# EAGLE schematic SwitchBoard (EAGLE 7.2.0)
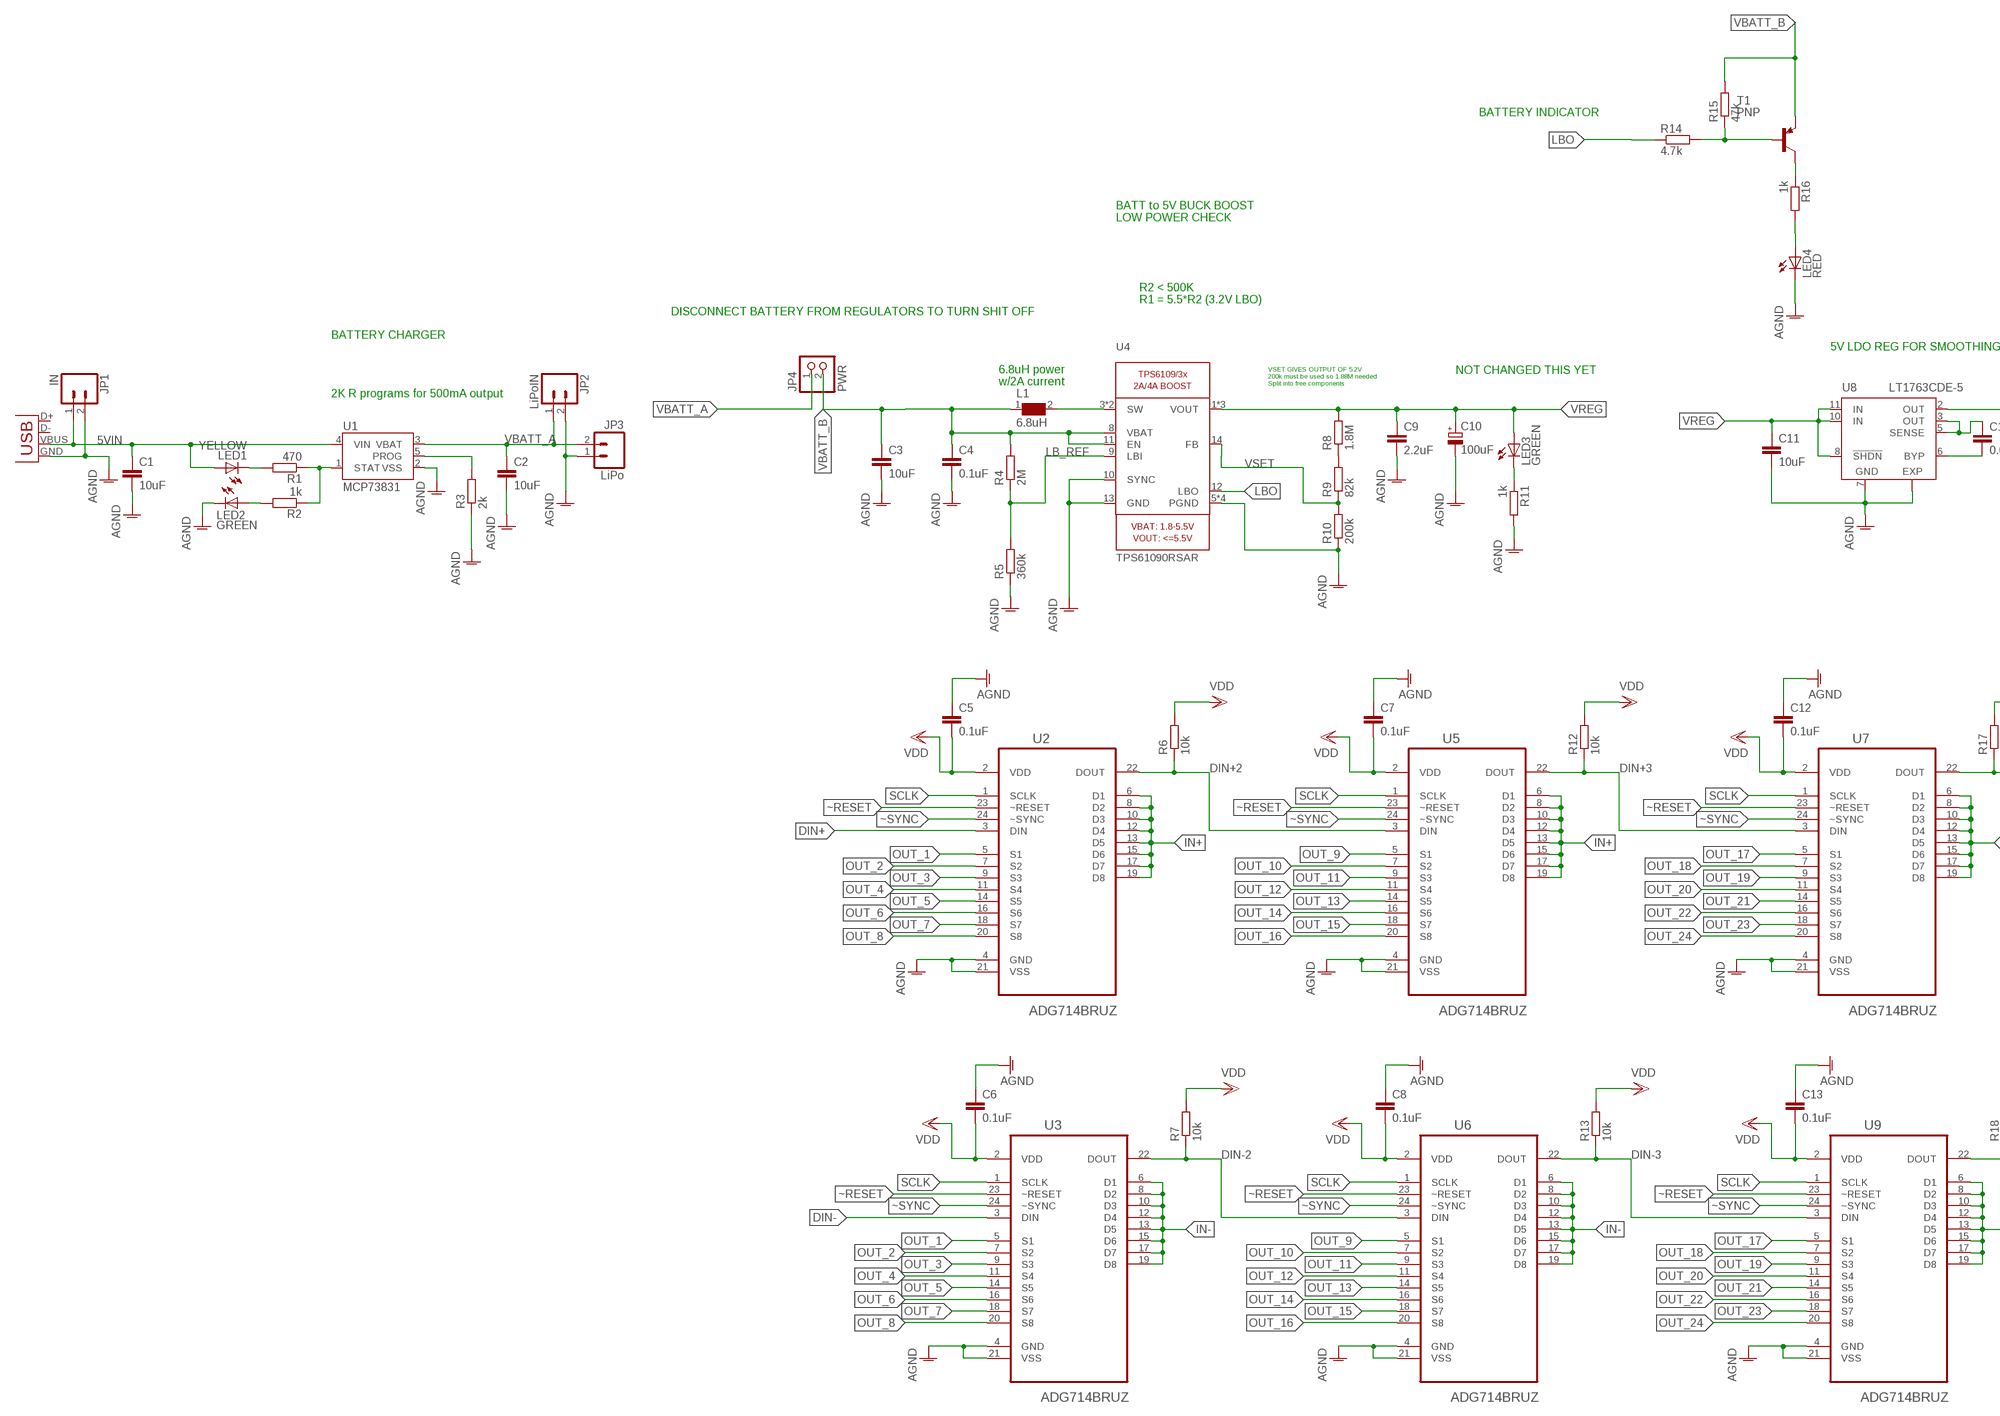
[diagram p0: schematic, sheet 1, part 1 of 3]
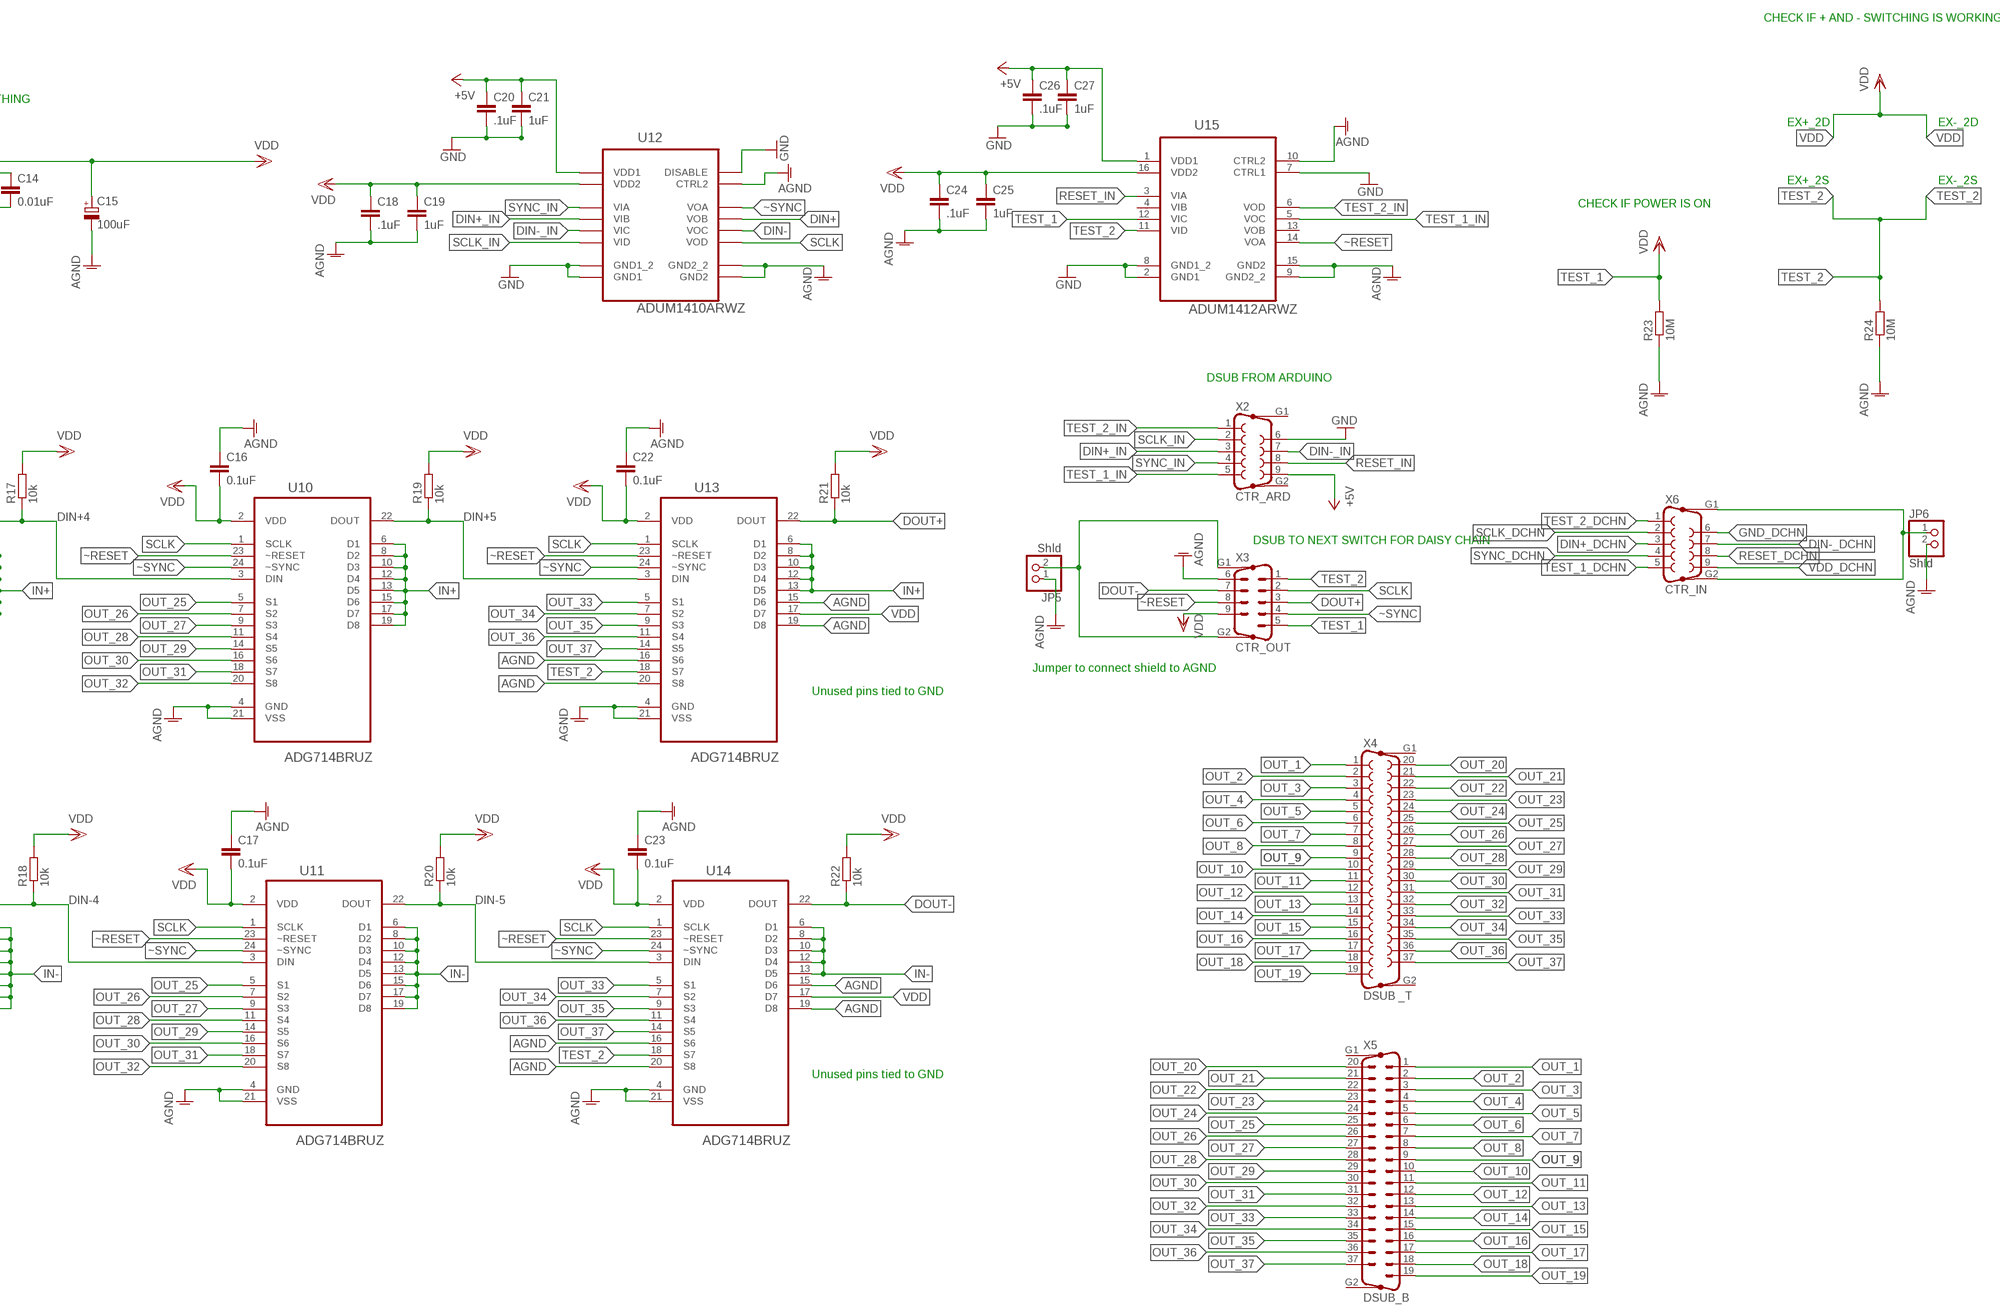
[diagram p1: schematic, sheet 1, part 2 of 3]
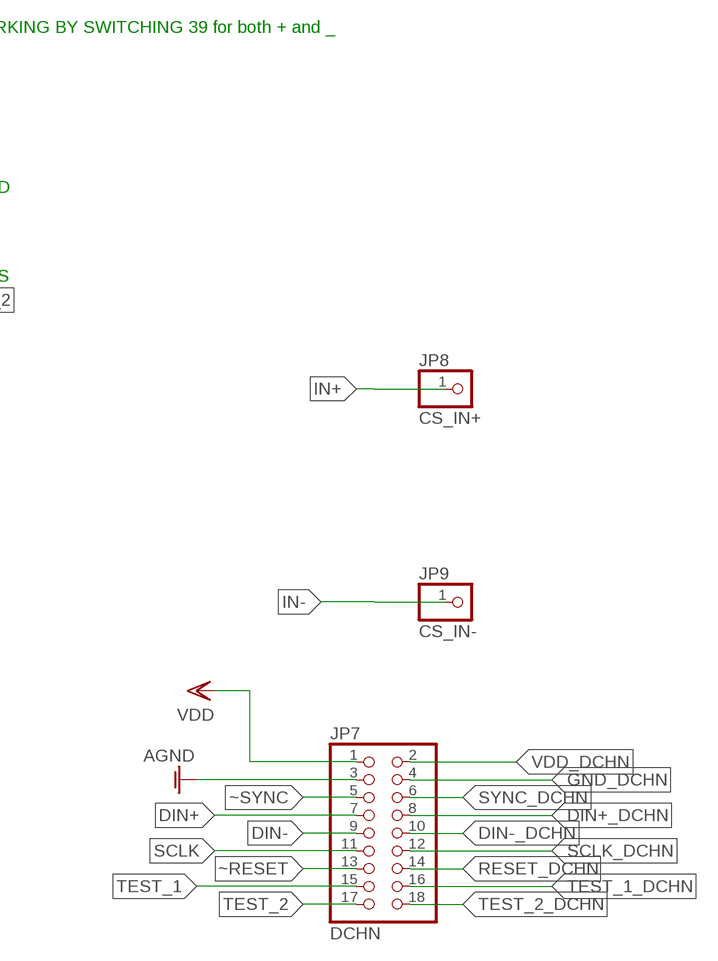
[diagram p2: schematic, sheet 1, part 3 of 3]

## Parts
C1  10uF  C-EUC0805  [C0805]
C2  10uF  C-EUC0805  [C0805]
C3  10uF  C-EUC0805  [C0805]
C4  0.1uF  C-EUC0805  [C0805]
C5  0.1uF  C-EUC0805  [C0805]
C6  0.1uF  C-EUC0805  [C0805]
C7  0.1uF  C-EUC0805  [C0805]
C8  0.1uF  C-EUC0805  [C0805]
C9  2.2uF  C-EUC0805  [C0805]
C10  100uF  CPOL-EUCT6032  [CT6032]
C11  10uF  C-EUC0805  [C0805]
C12  0.1uF  C-EUC0805  [C0805]
C13  0.1uF  C-EUC0805  [C0805]
C14  0.01uF  C-EUC0805  [C0805]
C15  100uF  CPOL-EUCT6032  [CT6032]
C16  0.1uF  C-EUC0805  [C0805]
C17  0.1uF  C-EUC0805  [C0805]
C18  .1uF  C-EUC0805  [C0805]
C19  1uF  C-EUC0805  [C0805]
C20  .1uF  C-EUC0805  [C0805]
C21  1uF  C-EUC0805  [C0805]
C22  0.1uF  C-EUC0805  [C0805]
C23  0.1uF  C-EUC0805  [C0805]
C24  .1uF  C-EUC0805  [C0805]
C25  1uF  C-EUC0805  [C0805]
C26  .1uF  C-EUC0805  [C0805]
C27  1uF  C-EUC0805  [C0805]
JP1  IN  M02PTH  [1X02]
JP2  LiPoIN  M02PTH  [1X02]
JP3  LiPo  M02-JST-2MM-SMT  [JST-2-SMD]
JP4  PWR  PINHD-1X2  [1X02]
JP5  Shld  PINHD-1X2  [1X02]
JP6  Shld  PINHD-1X2  [1X02]
JP7  DCHN  PINHD-2X9  [2X09]
JP8  CS_IN+  PINHD-1X1  [1X01]
JP9  CS_IN-  PINHD-1X1  [1X01]
L1  6.8uH  WE-PD-7447779006_7332/7345_PLASTIC_BASE  [WE-PD_7332/7345_PLASTIC_BASE]
LED1  YELLOW  LEDSML0805  [SML0805]
LED2  GREEN  LEDSML0805  [SML0805]
LED3  GREEN  LEDSML0805  [SML0805]
LED4  RED  LEDSML0805  [SML0805]
R1  470  R-EU_M0805  [M0805]
R2  1k  R-EU_M0805  [M0805]
R3  2k  R-EU_M0805  [M0805]
R4  2M  R-EU_M0805  [M0805]
R5  360k  R-EU_M0805  [M0805]
R6  10k  R-EU_M0805  [M0805]
R7  10k  R-EU_M0805  [M0805]
R8  1.8M  R-EU_M0805  [M0805]
R9  82k  R-EU_M0805  [M0805]
R10  200k  R-EU_M0805  [M0805]
R11  1k  R-EU_M0805  [M0805]
R12  10k  R-EU_M0805  [M0805]
R13  10k  R-EU_M0805  [M0805]
R14  4.7k  R-EU_M0805  [M0805]
R15  47k  R-EU_M0805  [M0805]
R16  1k  R-EU_M0805  [M0805]
R17  10k  R-EU_M0805  [M0805]
R18  10k  R-EU_M0805  [M0805]
R19  10k  R-EU_M0805  [M0805]
R20  10k  R-EU_M0805  [M0805]
R21  10k  R-EU_M0805  [M0805]
R22  10k  R-EU_M0805  [M0805]
R23  10M  R-EU_M0805  [M0805]
R24  10M  R-EU_M0805  [M0805]
T1  PNP  BC807-40-PNP-SOT23-BEC  [SOT23-BEC]
U1  MCP73831  [SOT23-5]
U2  ADG714BRUZ  [SOP65P640X120-24N]
U3  ADG714BRUZ  [SOP65P640X120-24N]
U4  TPS61090RSAR  VREG_TPS6103XSPARKFUNVERSION  [QFN16-4X4]
U5  ADG714BRUZ  [SOP65P640X120-24N]
U6  ADG714BRUZ  [SOP65P640X120-24N]
U7  ADG714BRUZ  [SOP65P640X120-24N]
U8  LT1763CDE-5  [DFN12]
U9  ADG714BRUZ  [SOP65P640X120-24N]
U10  ADG714BRUZ  [SOP65P640X120-24N]
U11  ADG714BRUZ  [SOP65P640X120-24N]
U12  ADUM1410ARWZ  [SOIC127P1032X265-16N]
U13  ADG714BRUZ  [SOP65P640X120-24N]
U14  ADG714BRUZ  [SOP65P640X120-24N]
U15  ADUM1412ARWZ  [SOIC127P1032X265-16N]
X1  USB-MICROB  [USB-MICROB]
X2  CTR_ARD  F09HP  [F09HP]
X3  CTR_OUT  M09HP  [M09HP]
X4  DSUB _T  F37HP  [F37HP]
X5  DSUB_B  M37HP  [M37HP]
X6  CTR_IN  F09HP  [F09HP]

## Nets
5VIN: C1.1 JP1.1 LED1.A U1.4(VIN) X1.VBUS
+5V: C20.1 C21.1 C26.1 C27.1 U12.1(VDD1) U15.1(VDD1) X2.9
AGND: C1.2 C2.2 C3.2 C4.2 C5.1 C6.1 C7.1 C8.1 C9.2 C10.- C11.2 C12.1 C13.1 C15.- C16.1 C17.1 C18.2 C19.2 C22.1 C23.1 C24.2 C25.2 JP1.2 JP2.2 JP3.1 JP5.1 JP6.2 JP7.3 LED2.C LED4.C R3.1 R5.1 R10.1 R11.2 R23.1 R24.1 U1.2(VSS) U2.4(GND) U2.21(VSS) U3.4(GND) U3.21(VSS) U4.5(PGND) U4.6(PGND) U4.7(PGND) U4.10(SYNC) U4.13(GND) U4.EXP(PGND) U5.4(GND) U5.21(VSS) U6.4(GND) U6.21(VSS) U7.4(GND) U7.21(VSS) U8.7(GND) U8.EXP U9.4(GND) U9.21(VSS) U10.4(GND) U10.21(VSS) U11.4(GND) U11.21(VSS) U12.9(GND2_2) U12.10(CTRL2) U12.15(GND2) U13.4(GND) U13.15(D6) U13.16(S6) U13.19(D8) U13.20(S8) U13.21(VSS) U14.4(GND) U14.15(D6) U14.16(S6) U14.19(D8) U14.20(S8) U14.21(VSS) U15.9(GND2_2) U15.10(CTRL2) U15.15(GND2) X1.GND X3.6
CHRG: LED1.C R1.2
DIN+: JP7.7 U2.3(DIN) U12.13(VOB)
DIN+2: R6.1 U2.22(DOUT) U5.3(DIN)
DIN+3: R12.1 U5.22(DOUT) U7.3(DIN)
DIN+4: R17.1 U7.22(DOUT) U10.3(DIN)
DIN+5: R19.1 U10.22(DOUT) U13.3(DIN)
DIN+_DCHN: JP7.8 X6.3
DIN+_IN: U12.4(VIB) X2.3
DIN-: JP7.9 U3.3(DIN) U12.12(VOC)
DIN-2: R7.1 U3.22(DOUT) U6.3(DIN)
DIN-3: R13.1 U6.22(DOUT) U9.3(DIN)
DIN-4: R18.1 U9.22(DOUT) U11.3(DIN)
DIN-5: R20.1 U11.22(DOUT) U14.3(DIN)
DIN-_DCHN: JP7.10 X6.7
DIN-_IN: U12.5(VIC) X2.7
DOUT+: R21.1 U13.22(DOUT) X3.3
DOUT-: R22.1 U14.22(DOUT) X3.7
GND: C20.2 C21.2 C26.2 C27.2 U12.2(GND1_2) U12.7(DISABLE) U12.8(GND1) U15.2(GND1) U15.7(CTRL1) U15.8(GND1_2) X2.6
GND_DCHN: JP7.4 X6.6
IN+: JP8.1 U2.6(D1) U2.8(D2) U2.10(D3) U2.12(D4) U2.13(D5) U2.15(D6) U2.17(D7) U2.19(D8) U5.6(D1) U5.8(D2) U5.10(D3) U5.12(D4) U5.13(D5) U5.15(D6) U5.17(D7) U5.19(D8) U7.6(D1) U7.8(D2) U7.10(D3) U7.12(D4) U7.13(D5) U7.15(D6) U7.17(D7) U7.19(D8) U10.6(D1) U10.8(D2) U10.10(D3) U10.12(D4) U10.13(D5) U10.15(D6) U10.17(D7) U10.19(D8) U13.6(D1) U13.8(D2) U13.10(D3) U13.12(D4) U13.13(D5)
IN-: JP9.1 U3.6(D1) U3.8(D2) U3.10(D3) U3.12(D4) U3.13(D5) U3.15(D6) U3.17(D7) U3.19(D8) U6.6(D1) U6.8(D2) U6.10(D3) U6.12(D4) U6.13(D5) U6.15(D6) U6.17(D7) U6.19(D8) U9.6(D1) U9.8(D2) U9.10(D3) U9.12(D4) U9.13(D5) U9.15(D6) U9.17(D7) U9.19(D8) U11.6(D1) U11.8(D2) U11.10(D3) U11.12(D4) U11.13(D5) U11.15(D6) U11.17(D7) U11.19(D8) U14.6(D1) U14.8(D2) U14.10(D3) U14.12(D4) U14.13(D5)
LB_REF: R4.1 R5.2 U4.9(LBI)
LBO: R14.1 U4.12(LBO)
N$3: C14.1 U8.3(OUT) U8.5(SENSE)
N$4: C14.2 U8.6(BYP)
N$5: LED2.A R2.2
N$6: R8.1 R9.2
N$7: LED3.C R11.1
N$8: R16.1 T1.C
N$9: LED4.A R16.2
N$10: JP5.2 X3.G1 X3.G2
N$11: R14.2 R15.1 T1.B
N$12: JP6.1 X6.G1 X6.G2
OUT_1: U2.5(S1) U3.5(S1) X4.1 X5.1
OUT_2: U2.7(S2) U3.7(S2) X4.2 X5.2
OUT_3: U2.9(S3) U3.9(S3) X4.3 X5.3
OUT_4: U2.11(S4) U3.11(S4) X4.4 X5.4
OUT_5: U2.14(S5) U3.14(S5) X4.5 X5.5
OUT_6: U2.16(S6) U3.16(S6) X4.6 X5.6
OUT_7: U2.18(S7) U3.18(S7) X4.7 X5.7
OUT_8: U2.20(S8) U3.20(S8) X4.8 X5.8
OUT_9: U5.5(S1) U6.5(S1) X4.9 X5.9
OUT_10: U5.7(S2) U6.7(S2) X4.10 X5.10
OUT_11: U5.9(S3) U6.9(S3) X4.11 X5.11
OUT_12: U5.11(S4) U6.11(S4) X4.12 X5.12
OUT_13: U5.14(S5) U6.14(S5) X4.13 X5.13
OUT_14: U5.16(S6) U6.16(S6) X4.14 X5.14
OUT_15: U5.18(S7) U6.18(S7) X4.15 X5.15
OUT_16: U5.20(S8) U6.20(S8) X4.16 X5.16
OUT_17: U7.5(S1) U9.5(S1) X4.17 X5.17
OUT_18: U7.7(S2) U9.7(S2) X4.18 X5.18
OUT_19: U7.9(S3) U9.9(S3) X4.19 X5.19
OUT_20: U7.11(S4) U9.11(S4) X4.20 X5.20
OUT_21: U7.14(S5) U9.14(S5) X4.21 X5.21
OUT_22: U7.16(S6) U9.16(S6) X4.22 X5.22
OUT_23: U7.18(S7) U9.18(S7) X4.23 X5.23
OUT_24: U7.20(S8) U9.20(S8) X4.24 X5.24
OUT_25: U10.5(S1) U11.5(S1) X4.25 X5.25
OUT_26: U10.7(S2) U11.7(S2) X4.26 X5.26
OUT_27: U10.9(S3) U11.9(S3) X4.27 X5.27
OUT_28: U10.11(S4) U11.11(S4) X4.28 X5.28
OUT_29: U10.14(S5) U11.14(S5) X4.29 X5.29
OUT_30: U10.16(S6) U11.16(S6) X4.30 X5.30
OUT_31: U10.18(S7) U11.18(S7) X4.31 X5.31
OUT_32: U10.20(S8) U11.20(S8) X4.32 X5.32
OUT_33: U13.5(S1) U14.5(S1) X4.33 X5.33
OUT_34: U13.7(S2) U14.7(S2) X4.34 X5.34
OUT_35: U13.9(S3) U14.9(S3) X4.35 X5.35
OUT_36: U13.11(S4) U14.11(S4) X4.36 X5.36
OUT_37: U13.14(S5) U14.14(S5) X4.37 X5.37
PROG: R3.2 U1.5(PROG)
RESET_DCHN: JP7.14 X6.8
RESET_IN: U15.3(VIA) X2.8
SCLK: JP7.11 U2.1(SCLK) U3.1(SCLK) U5.1(SCLK) U6.1(SCLK) U7.1(SCLK) U9.1(SCLK) U10.1(SCLK) U11.1(SCLK) U12.11(VOD) U13.1(SCLK) U14.1(SCLK) X3.2
SCLK_DCHN: JP7.12 X6.2
SCLK_IN: U12.6(VID) X2.2
STAT: R1.1 R2.1 U1.1(STAT)
SW: L1.2 U4.3(SW) U4.4(SW)
SYNC_DCHN: JP7.6 X6.4
SYNC_IN: U12.3(VIA) X2.4
TEST_1: JP7.15 R23.2 U15.12(VIC) X3.5 ; supply symbol labelled VDD
TEST_1_DCHN: JP7.16 X6.5
TEST_1_IN: U15.5(VOC) X2.5
TEST_2: JP7.17 R24.2 U13.18(S7) U14.18(S7) U15.11(VID) X3.1
TEST_2_DCHN: JP7.18 X6.1
TEST_2_IN: U15.6(VOD) X2.1
VBATT_A: C2.1 JP2.1 JP3.2 JP4.1 U1.3(VBAT)
VBATT_B: C3.1 C4.1 JP4.2 L1.1 R4.2 R15.2 T1.E U4.8(VBAT) U4.11(EN)
VDD: C5.2 C6.2 C7.2 C8.2 C12.2 C13.2 C15.+ C16.2 C17.2 C18.1 C19.1 C22.2 C23.2 C24.1 C25.1 JP7.1 R6.2 R7.2 R12.2 R13.2 R17.2 R18.2 R19.2 R20.2 R21.2 R22.2 U2.2(VDD) U3.2(VDD) U5.2(VDD) U6.2(VDD) U7.2(VDD) U8.2(OUT) U9.2(VDD) U10.2(VDD) U11.2(VDD) U12.16(VDD2) U13.2(VDD) U13.17(D7) U14.2(VDD) U14.17(D7) U15.16(VDD2) X3.9
VDD_DCHN: JP7.2 X6.9
VREG: C9.1 C10.+ C11.1 LED3.A R8.2 U4.1(VOUT) U4.15(VOUT) U4.16(VOUT) U8.8(!SHDN) U8.10(IN) U8.11(IN)
VSET: R9.1 R10.2 U4.14(FB)
~RESET: JP7.13 U2.23(~RESET) U3.23(~RESET) U5.23(~RESET) U6.23(~RESET) U7.23(~RESET) U9.23(~RESET) U10.23(~RESET) U11.23(~RESET) U13.23(~RESET) U14.23(~RESET) U15.14(VOA) X3.8
~SYNC: JP7.5 U2.24(~SYNC) U3.24(~SYNC) U5.24(~SYNC) U6.24(~SYNC) U7.24(~SYNC) U9.24(~SYNC) U10.24(~SYNC) U11.24(~SYNC) U12.14(VOA) U13.24(~SYNC) U14.24(~SYNC) X3.4
Unconnected: U15.4(VIB) U15.13(VOB) X1.D+ X1.D- X2.G1 X2.G2 X4.G1 X4.G2 X5.G1 X5.G2

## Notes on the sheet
- BATTERY INDICATOR
- BATT to 5V BUCK BOOST
  LOW POWER CHECK
- CHECK IF + AND - SWITCHING IS WORKING BY SWITCHING 39 for both + and _
- R2 < 500K
  R1 = 5.5*R2 (3.2V LBO)
- DISCONNECT BATTERY FROM REGULATORS TO TURN SHIT OFF
- BATTERY CHARGER
- 5V LDO REG FOR SMOOTHING
- NOT CHANGED THIS YET | EX+_2D | EX-_2D
- 6.8uH power
  w/2A current
- VSET GIVES OUTPUT OF 5.2V
  200k must be used so 1.88M needed
  Split into free components
- 2K R programs for 500mA output
- EX+_2S | EX-_2S
- CHECK IF POWER IS ON
- DSUB FROM ARDUINO
- DSUB TO NEXT SWITCH FOR DAISY CHAIN
- Jumper to connect shield to AGND
- Unused pins tied to GND
- Unused pins tied to GND

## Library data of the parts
C1-C9 C11-C14 C16-C27 = resistor:C-EU: CAPACITOR, European symbol
C10 C15 = rcl:CPOL-EU: POLARIZED CAPACITOR, European symbol
JP1-JP3 = SparkFun:M02: Header 2
JP4-JP6 = pinhead:PINHD-1X2: PIN HEADER
JP7 = pinhead:PINHD-2X9: PIN HEADER
JP8 JP9 = pinhead:PINHD-1X1: PIN HEADER
L1 = WE-PD:WE-PD: SMD-Shielded Power Inductors WE-PD; MPN: 7447779006; OC_FARNELL: 1635987; OC_NEWARK: 08P2857; PACKAGE: 7345; SUPPLIER: Wuerth Elektronik
LED1-LED4 = led:LED: LED
R1-R24 = rcl:R-EU_: RESISTOR, European symbol
T1 = transistor:*-PNP-: PNP Transistror
U1 = SparkFun-PowerIC:MCP73831: Miniature single cell, fully integrated Li-Ion, Li-polymer charge management controller http://ww1.microchip.com/downloads/en/DeviceDoc/20001984g.pdf IC-09995; PROD_ID: IC-09995
U2 U3 U5-U7 U9-U11 U13 U14 = Analog Devices_By_element14_Batch_1:ADG714BRUZ: CMOS, Low Voltage Serially Controlled, Octal SPST Switches; MPN: ADG714BRUZ; OC_FARNELL: 9604367; OC_NEWARK: 59K1531; PACKAGE: TSSOP-24; SUPPLIER: Analog Devices
U4 = Adafruit PowerBoost 500C:VREG_TPS6103X: TPS6103x 4A Boost - 1.8-5.5V Input, Adjustable Output to 5.5V
U8 = linear-technology:LT1763: 500mA, Low Noise, LDO Micropower Regulators Source: http://cds.linear.com/docs/Datasheet/1763ff.pdf; MPN: LT1763CDE-5; OC_FARNELL: 1556468; OC_NEWARK: 57M6035
U12 = ADI-Phase-2:ADUM1410ARWZ: ISOLATOR, DGTL, 4CHAN; MPN: ADUM1410ARWZ; OC_FARNELL: 2067770; OC_NEWARK: 73T8174; PACKAGE: 16-Lead SOIC_W; SUPPLIER: Analog Devices
U15 = ADUM1412JAMES:ADUM1412ARWZ: IC, DIG ISOLATOR; MPN: ADUM1412ARWZ; OC_FARNELL: 2377152; PACKAGE: 16-Lead SOIC_W; SUPPLIER: Analog Devices
X1 = SparkFun:USB: USB Connectors USB-B-PTH is fully proven SKU : PRT-00139 USB-miniB is fully proven SKU : PRT-00587 USB-A-PCB is untested. USB-A-H is throughly reviewed, but untested. Spark Fun Electronics SKU : PRT-00437 USB-B-SMT is throughly reviewed, but untested. Needs silkscreen touching up. USB-A-S has not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
X2 X6 = con-subd:F09HP: SUB-D; OC_FARNELL: unknown; OC_NEWARK: unknown
X3 = con-subd:M09HP: SUB-D; OC_FARNELL: unknown; OC_NEWARK: unknown
X4 = con-subd:F37HP: SUB-D; OC_FARNELL: unknown; OC_NEWARK: unknown
X5 = con-subd:M37HP: SUB-D; OC_FARNELL: unknown; OC_NEWARK: unknown

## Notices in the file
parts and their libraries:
SparkFun-PowerIC: Licensing: Creative Commons ShareAlike 4.0 International - https://creativecommons.org/licenses/by-sa/4.0
